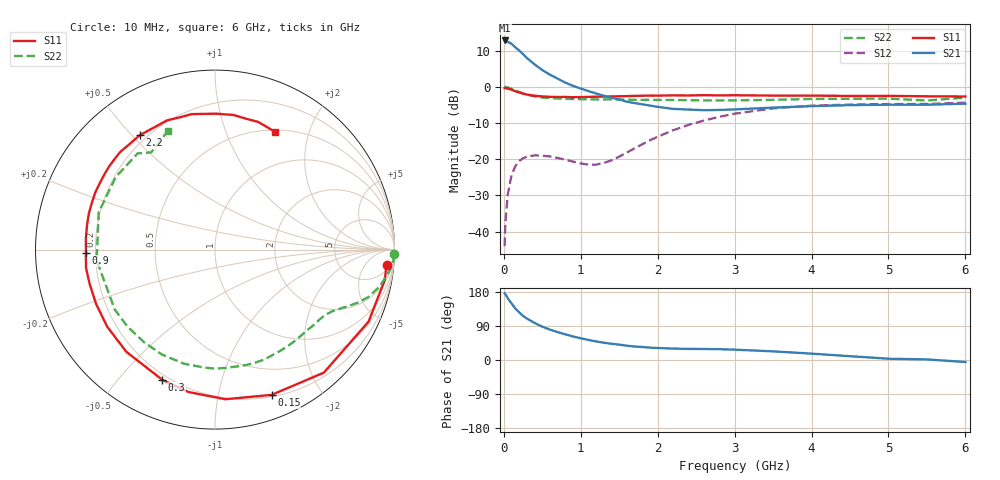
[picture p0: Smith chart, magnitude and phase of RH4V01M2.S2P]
! SIEMENS Small Signal Semiconductors
! BFR106
! Si NPN RF Bipolar Junction Transistor in SOT23
! VCE = 4 V  IC = 1.2 mA
! Common Emitter S-Parameters:  August  1996
# GHz  S  MA  R  50
!  f  S11  S21  S12  S22
! GHz  MAG  ANG  MAG  ANG  MAG  ANG  MAG  ANG
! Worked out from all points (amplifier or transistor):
!   36 points, 10 MHz to 6 GHz, reference 50 ohm
!   highest |S21| = 12.8 dB at 10 MHz (marker M1)
!   |S21| within 3 dB of that: start of sweep to 210.3 MHz
!   unconditionally stable (mu >= 1): 842.3 MHz to 1.897 GHz; 3.123 GHz to end of sweep
!   at 250 MHz: K = 0.27, MSG = 14.4 dB, |S12| = -19.7 dB
!   at 1.4 GHz: K = 1.38, MAG = 4.9 dB, |S12| = -20.3 dB
!   at 6 GHz: K = 1.02, MAG = -1.0 dB, |S12| = -4.4 dB
!   S11 on the Smith chart (normalised r, x): 10 MHz: 9, -19; 150 MHz: 0.22, -1.44; 300 MHz: 0.18, -0.66; 900 MHz: 0.16, -0.01; 2.2 GHz: 0.17, +0.53; 6 GHz: 0.52, +1.50
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0.01  0.96 -5.0  4.376 176.1  0.0063 89.2  0.9989 -1.5
0.02  0.9609 -10.2  4.358 173.6  0.0132 83.9  0.9987 -2.9
0.05  0.9452 -25.1  4.202 163.3  0.0323 75.6  0.9803 -6.8
0.1  0.9153 -48.5  3.935 149.3  0.0602 63.7  0.9408 -12.6
0.15  0.8687 -68.7  3.519 135.6  0.0805 52.5  0.894 -17.2
0.2  0.8357 -86.0  3.173 125.6  0.0943 44.4  0.85 -20.3
0.25  0.8072 -100.5  2.824 116.2  0.1034 37.6  0.8091 -22.8
0.3  0.7823 -112.1  2.504 109.3  0.1086 33.0  0.7803 -24.6
0.4  0.7539 -130.9  2.044 97.7  0.1131 25.4  0.7385 -27.7
0.5  0.7383 -144.5  1.706 87.9  0.1121 21.2  0.7133 -30.7
0.7  0.7239 -164.7  1.296 73.5  0.1042 18.2  0.6915 -37.6
0.9  0.7196 -178.6  1.032 62.2  0.0927 22.3  0.6786 -44.7
1.1  0.7263 168.8  0.873 53.0  0.0843 34.3  0.6736 -52.9
1.3  0.7341 159.0  0.753 45.6  0.089 51.1  0.6693 -61.5
1.6  0.7452 145.7  0.623 37.7  0.1237 69.5  0.6661 -75.1
2.2  0.7628 123.4  0.496 30.2  0.2514 71.6  0.6587 -105.3
2.8  0.7624 104.7  0.48 28.5  0.3853 57.9  0.6494 -138.7
3.5  0.7573 89.6  0.517 22.8  0.5045 39.5  0.6622 -174.9
4.5  0.7494 76.4  0.559 10.0  0.5695 16.9  0.6852 143.8
5  0.7508 71.4  0.567 3.4  0.5779 8.5  0.6877 128.8
5.5  0.7408 66.4  0.566 1.5  0.5804 4.5  0.648 123.3
6  0.7363 63.1  0.586 -5.3  0.6046 -3.4  0.7108 111.7
